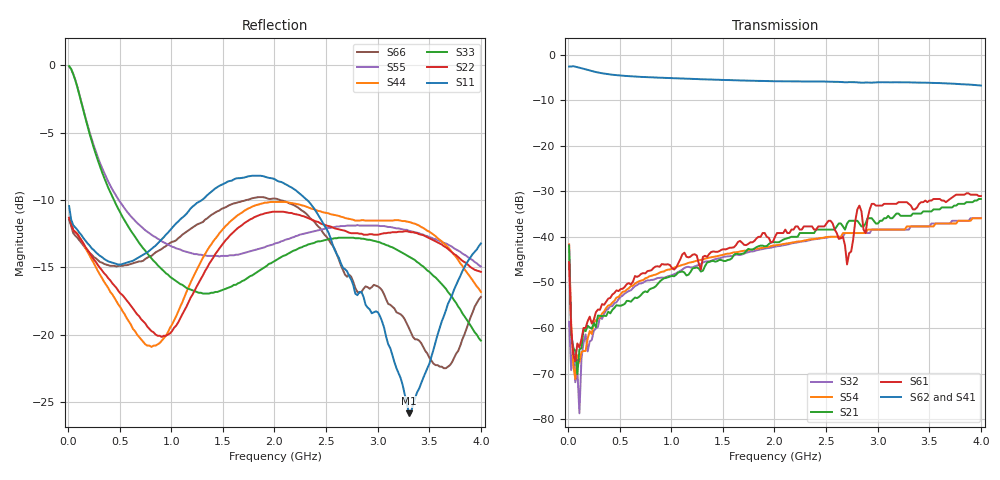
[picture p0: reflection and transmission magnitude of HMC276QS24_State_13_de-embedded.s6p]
! Hittite Microwave Corporation
! 20 Alpha Road
! Chelmsford, MA 01824
! Tel: 978-250-3343
! Fax: 978-250-3373
! Device: HMC276QS24, 0.7-3.0 GHz, GaAS MMIC 4x2 Switch Matrix in 24-lead QSOP package
! Misc: Data was de-embedded to package pins.
!  Port 1 = OP1
!  Port 2 = VL
!  Port 3 = VH
!  Port 4 = HH
!  Port 5 = HL
!  Port 6 = OP2
!  Vdd = +5 V
!  Vctl = 0 V[Logic 0] / +5 V[Logic 1]
!  State 13,  HH to OP1,  VL to OP2
!  Control Lines (Logic)
!  HV 1 = 1, Tone 1 = 1
!  HV 2 = 0, Tone 2 = 0
!  Data reformated to new Touchstone file format - Wed Jan 10 15:57:24 2007
# MHz S DB R 50
! 6 Port Network Data
! freq  dbS11  angS11  dbS12  angS12  dbS13  angS13  dbS14  angS14
!  dbS15  angS15  dbS16  angS16
!  dbS21  angS21  dbS22  angS22
!  dbS23  angS23  dbS24  angS24  dbS25  angS25  dbS26  angS26
!  dbS31  angS31  dbS32  angS32  dbS33  angS33  dbS34  angS34
!  dbS35  angS35  dbS36  angS36
!  dbS41  angS41  dbS42  angS42
!  dbS43  angS43  dbS44  angS44  dbS45  angS45  dbS46  angS46
!  dbS51  angS51  dbS52  angS52  dbS53  angS53  dbS54  angS54
!  dbS55  angS55  dbS56  angS56
!  dbS61  angS61  dbS62  angS62
!  dbS63  angS63  dbS64  angS64  dbS65  angS65  dbS66  angS66
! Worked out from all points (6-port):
!   201 points, 10 MHz to 4 GHz, reference 50 ohm
!   strongest paths, dB at 10 MHz, 1.008 GHz, 2.005 GHz, 3.002 GHz, 4 GHz:
!     S62: -2.7, -5.2, -5.9, -6.1, -6.8
!     S41: -2.9, -5.3, -6.1, -6.2, -7.0
!     S61: -45.6, -46.9, -40.0, -33.2, -31.1
!     S21: -41.9, -48.6, -41.2, -37.1, -31.7
!     S54: -41.7, -47.0, -41.9, -38.4, -35.9
!     S32: -58.6, -48.4, -42.2, -38.4, -35.9
!   lowest |S11| = -25.8 dB at 3.302 GHz (marker M1), VSWR 1.11, Z = 54.2 + j3.25 ohm
!   |S11| at or under -10 dB: start of sweep to 1.298 GHz; 2.315 GHz to end of sweep
